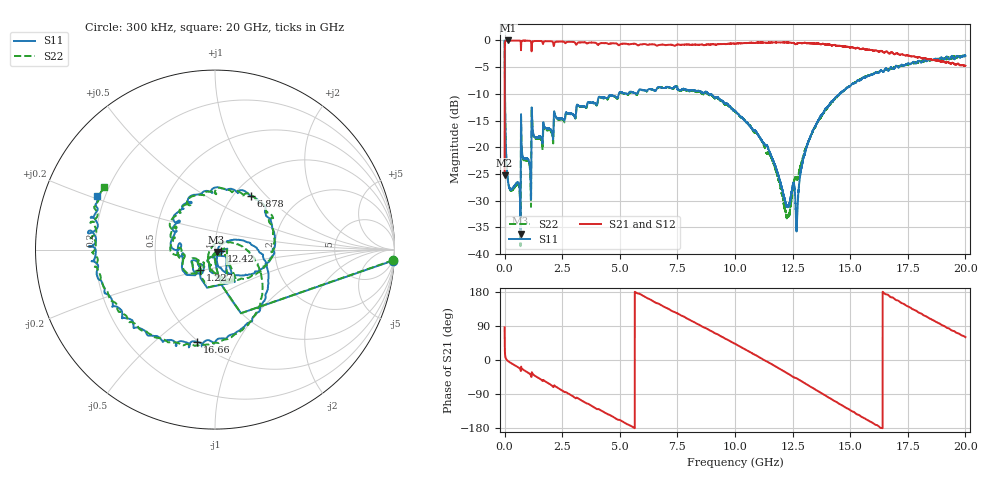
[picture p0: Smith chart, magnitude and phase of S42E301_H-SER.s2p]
!{S42E301}
!Johanson Technology Inc.
!www.johansontechnology.com
!Test Board Conditions:
!Substrate Type  RO4350B
!Substrate Thickness  50 mil
!Substrate Dk  3.66
!TL Type: GCPW
!TL Trace Width  60 mil
!TL Gap  10 mil
!Electrode orientation  Horizontal
!DUT TOPOLOGY	SERIES
!Mounting Pad LxW  14x55 mil
! Created Wed Nov 25 22:10:22 2020
# khz S ma R 50
! 2 Port Network Data from SP1.SP block
! freq  magS11  angS11  magS21  angS21  magS12  angS12  magS22  angS22
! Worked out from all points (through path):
!   20001 points, 300 kHz to 20 GHz, reference 50 ohm
!   highest |S21| = -0.01 dB at 157.3 MHz (marker M1); lowest = -25.2 dB at 300 kHz (marker M2)
!   group delay of S21, straight-line fit = 92.2 ps
!   lowest |S11| = -36.2 dB at 690.3 MHz (marker M3), VSWR 1.03, Z = 50.8 - j1.33 ohm
!   |S11| at or under -10 dB: 16.56 MHz to 4.96 GHz (4.943 GHz wide, 199 % of centre); 5.311 GHz to 5.366 GHz (54.39 MHz wide, 1.02 % of centre); 8.846 GHz to 14.54 GHz (5.696 GHz wide, 48.7 % of centre)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
!   |S22| runs from -38.5 to 0.0 dB; largest |S21 - S12| = 0.016
!   S11 on the Smith chart (normalised r, x): 300 kHz: 4, -32; 1.227 GHz: 0.82, -0.19; 6.878 GHz: 1.19, +0.82; 12.42 GHz: 1.07, -0.02; 16.66 GHz: 0.49, -0.70; 20 GHz: 0.17, +0.21
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300  0.9927 -3.6  0.05468 86.1  0.05431 85.9  0.9946 -3.4
101300  0.06157 -89.6  0.996 -0.2  0.9972 -0.3  0.06142 -89.4
157300  0.0463 -92.9  0.9985 -3.3  0.9982 -3.3  0.04619 -92.4
690300  0.01555 -57.2  0.9857 -25.3  0.9861 -25.3  0.01193 -53.9
1227300  0.142 -126.3  0.9798 -37.5  0.9798 -37.4  0.1386 -125.1
2007300  0.1462 -154.1  0.9813 -65.4  0.9813 -65.4  0.141 -158.2
3334300  0.2416 158.9  0.9592 -106.6  0.9594 -106.6  0.2399 167.6
5198300  0.32 106.1  0.932 -165.1  0.9307 -165.2  0.317 105.7
6667300  0.3653 64.5  0.9006 149.1  0.9001 149.0  0.3635 58.6
6878300  0.3585 56.4  0.9119 141.9  0.9089 141.8  0.3576 49.3
8486300  0.3343 3.1  0.9139 91.5  0.9135 91.6  0.3291 1.2
1.00003e7  0.2194 -40.6  0.9322 42.8  0.9309 42.7  0.2159 -49.6
1.11943e7  0.1127 -71.7  0.9554 2.3  0.9537 2.3  0.1118 -100.2
1.22243e7  0.02872 -50.5  0.956 -33.5  0.9575 -33.5  0.02292 164.0
1.24243e7  0.03468 -12.2  0.9497 -40.9  0.9515 -41.0  0.03001 95.7
1.27043e7  0.02376 31.7  0.9367 -49.5  0.9358 -49.5  0.04946 39.4
1.33343e7  0.1346 23.6  0.9403 -72.5  0.9399 -72.5  0.1349 11.5
1.50403e7  0.3819 -42.5  0.8619 -134.2  0.8623 -134.0  0.3837 -48.5
1.66553e7  0.5247 -100.9  0.764 171.4  0.7623 170.6  0.539 -99.5
1.66673e7  0.5241 -101.9  0.7592 170.8  0.7637 170.0  0.5422 -99.7
1.82553e7  0.6464 -151.6  0.683 116.3  0.674 116.8  0.6456 -153.9
2e7  0.7185 155.6  0.5786 60.4  0.578 60.8  0.7183 150.4
